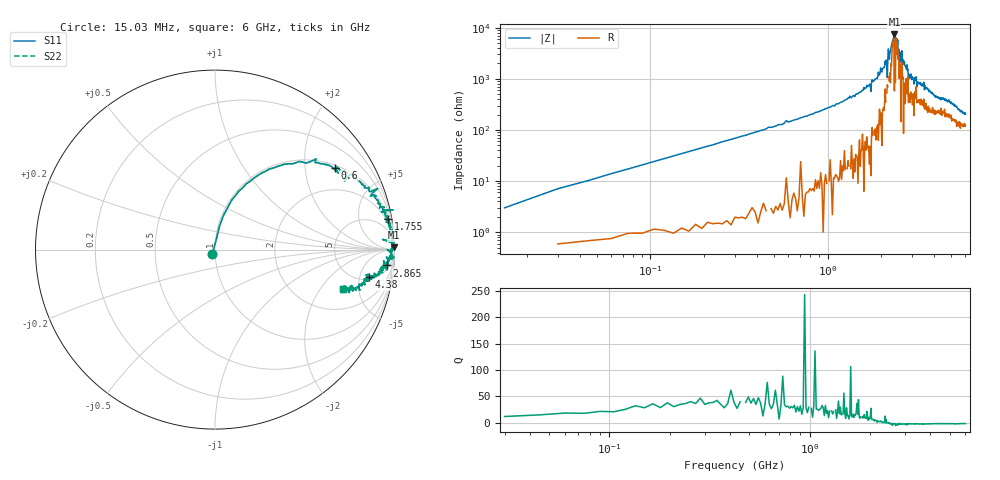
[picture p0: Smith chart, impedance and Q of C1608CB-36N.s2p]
!	Network	Analyzer	HP8753E.07.74:	Oct	30	2002	Serial	No.	JP38451487
!	Hewlett-Packard
!	28	Aug	2009	8:09:20
!	Frequency	S11	S21	S12	S22
#	HZ	S	RI	R	50
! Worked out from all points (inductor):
!   400 points, 15.03 MHz to 6 GHz, reference 50 ohm
!   read as one part in series: L = 36.7 nH near 45.03 MHz
!   highest |Z| = 7.37 kohm at 2.385 GHz (marker M1)
!   self-resonance near 2.415 GHz
!   S11 on the Smith chart (normalised r, x): 15.03 MHz: 0.97, -0.05; 600 MHz: 1.08, +2.87; 1.755 GHz: 1, +11; 2.865 GHz: 8, -18; 4.38 GHz: 5.57, -6.93; 6 GHz: 3.43, -3.32
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1.502992e7  -0.0152 -0.0251  1.02 0.0251  1.02 0.0251  -0.0152 -0.0251
6.00297e7  0.0264 0.135  0.974 -0.135  0.974 -0.135  0.0264 0.135
1.650292e8  0.133 0.326  0.867 -0.326  0.867 -0.326  0.133 0.326
6.00027e8  0.669 0.457  0.331 -0.457  0.331 -0.457  0.669 0.457
1.020025e9  0.875 0.313  0.125 -0.313  0.125 -0.313  0.875 0.313
1.755021e9  0.966 0.171  0.0343 -0.171  0.0343 -0.171  0.966 0.171
2.01002e9  0.989 0.0697  0.0114 -0.0697  0.0114 -0.0697  0.989 0.0697
2.145019e9  0.999 0.0429  0.000519 -0.0429  0.000519 -0.0429  0.999 0.0429
2.175019e9  0.933 0.057  0.0675 -0.057  0.0675 -0.057  0.933 0.057
2.205019e9  1 0.026  -0.0014 -0.026  -0.0014 -0.026  1 0.026
2.235019e9  0.983 0.0371  0.0165 -0.0371  0.0165 -0.0371  0.983 0.0371
2.385018e9  0.999 0.0135  0.00125 -0.0135  0.00125 -0.0135  0.999 0.0135
2.445018e9  0.972 -0.0109  0.028 0.0109  0.028 0.0109  0.972 -0.0109
2.490018e9  0.987 -0.0115  0.0129 0.0115  0.0129 0.0115  0.987 -0.0115
2.505017e9  0.96 -0.000671  0.0398 0.000671  0.0398 0.000671  0.96 -0.000671
2.625017e9  0.983 -0.0221  0.0167 0.0221  0.0167 0.0221  0.983 -0.0221
2.865016e9  0.958 -0.0884  0.0424 0.0884  0.0424 0.0884  0.958 -0.0884
3.015015e9  0.968 -0.0822  0.0318 0.0822  0.0318 0.0822  0.968 -0.0822
4.00501e9  0.887 -0.156  0.113 0.156  0.113 0.156  0.887 -0.156
4.380008e9  0.856 -0.152  0.144 0.152  0.144 0.152  0.856 -0.152
5.010005e9  0.832 -0.183  0.168 0.183  0.168 0.183  0.832 -0.183
6e9  0.711 -0.217  0.289 0.217  0.289 0.217  0.711 -0.217
